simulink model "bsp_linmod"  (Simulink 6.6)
settings: Solver=ode45  StartTime=0.0  StopTime=0.5  RelTol=1e-3

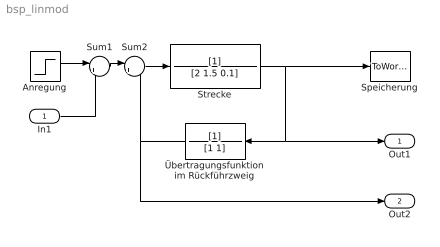
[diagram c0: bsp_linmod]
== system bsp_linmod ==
  In1 : Inport
  Anregung : Step  SampleTime=0
  Speicherung : ToWorkspace  VariableName=y  SampleTime=-1  SaveFormat=Array
  Strecke : TransferFcn  Denominator=[2 1.5 0.1]
  Sum1 : Sum  Inputs=|++
  Sum2 : Sum  Inputs=|+-
  Übertragungsfunktion im Rückführzweig : TransferFcn  Orientation=left  Denominator=[1 1]
  Out1 : Outport
  Out2 : Outport  Port=2
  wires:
  Sum2/1 -> Strecke/1
  Übertragungsfunktion im Rückführzweig/1 -> Sum2/2, Out2/1
  Strecke/1 -> Speicherung/1, Übertragungsfunktion im Rückführzweig/1, Out1/1
  Anregung/1 -> Sum1/1
  Sum1/1 -> Sum2/1
  In1/1 -> Sum1/2
